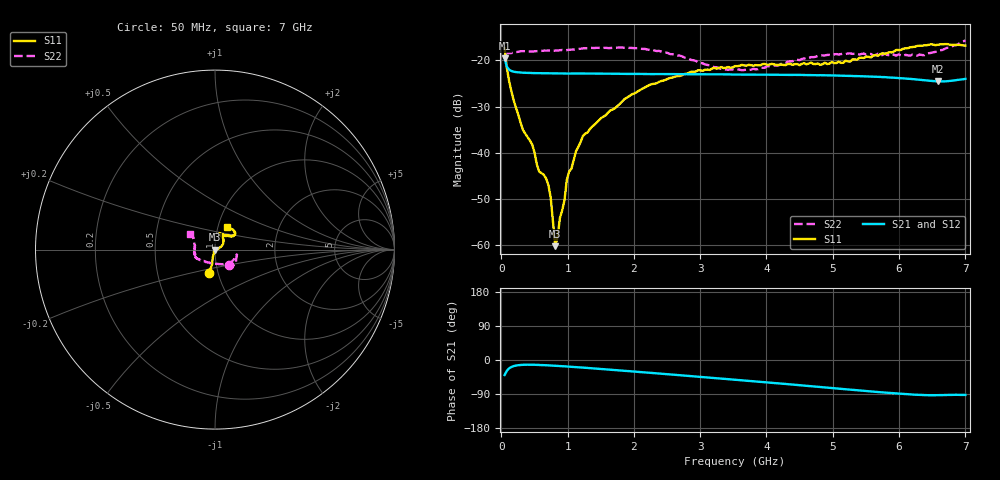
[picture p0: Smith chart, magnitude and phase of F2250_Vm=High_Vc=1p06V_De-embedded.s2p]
! Integrated Device Technology
! Corporate Headquarters
! 6024 Silver Creek Valley Road
! San Jose, CA 95138  USA
! Phone:  1-408-284-8200
! Toll Free:  1-800-223-1366
! Webpage:  http://www.idt.com/
! Timing and RF Division
! 515 Groton Road, Suite 102
! Westford, MA 01886-6024
! Device:  F2250
! Description: Voltage Variable RF Attenuator
! Frequency:  50.0 -  6000.00 MHz
! Package:  3x3 mm Thin QFN Plastic Package: 16 pin
! Ports:  2 RF, 3 DC
!  Pin  1  = GND
!  Pin  2  = NC
!  Pin  3  = RF1  = Port 1
!  Pin  4  = NC
!  Pin  5  = GND
!  Pin  6  = GND
!  Pin  7  = GND
!  Pin  8  = GND
!  Pin  9  = NC
!  Pin 10  = RF2  = Port 2
!  Pin 11  = NC
!  Pin 12  = GND
!  Pin 13  = GND
!  Pin 14  = VCNTRL
!  Pin 15  = VDD
!  Pin 16  = VMODE
! Vcntrl:  1.060 Volts
! Vmode:  +3.300 Volts
! Vdd:  +3.30  Volts
! Current:  1.329 mA
! Data:  The device was measured on a the F2250 evaluation board which has
!  individual transmission lines to the RF pins.  Data was collected
!  using a calibrated network analyzer.  The evaluation board was
!  de-embedded using a TRL calibration technique.
!  The reference plane is the edge of the package pin.
! Misc:  SN 10
!  Action Tracker AT0258
! Date Measured:  2014-11-26
! Date:  2015-10-15  MJV
! Note:
!  Integrated Device Technology supplies this data as a sample of measured
!  data at the package pin for this product.  Your particular data for this
!  product may vary.
!  Data was taken at 25 degrees C.
!  Integrated Device Technology reserves the right to change this data at anytime.
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# GHz S dB R 50
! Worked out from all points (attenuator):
!   201 points, 50 MHz to 7 GHz, reference 50 ohm
!   highest |S21| = -19.60 dB at 50 MHz (marker M1); lowest = -24.6 dB at 6.583 GHz (marker M2)
!   lowest |S11| = -60.2 dB at 814.5 MHz (marker M3), VSWR 1.00, Z = 50 - j0.0982 ohm
!   |S11| at or under -10 dB: start of sweep to end of sweep
!   |S22| runs from -22.2 to -15.7 dB; largest |S21 - S12| = 0.00029
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0.05  -17.37 -104.3  -19.60 -39.6  -19.60 -39.6  -18.87 -48.0
0.1195  -24.60 -103.5  -22.03 -21.8  -22.03 -21.8  -18.44 -18.2
0.29325  -33.58 -105.8  -22.64 -13.1  -22.63 -13.1  -18.03 -13.5
0.467  -38.21 -116.0  -22.75 -12.5  -22.74 -12.5  -18.09 -14.2
0.57125  -44.04 -115.3  -22.77 -13.0  -22.78 -13.1  -18.01 -16.4
0.71025  -46.92 -104.7  -22.80 -14.2  -22.79 -14.2  -17.89 -19.2
0.745  -49.63 -99.7  -22.81 -14.5  -22.80 -14.5  -17.87 -19.8
0.8145  -60.15 -88.2  -22.81 -15.2  -22.81 -15.2  -17.91 -21.5
0.84925  -58.21 -63.9  -22.83 -15.6  -22.83 -15.6  -17.87 -22.5
0.884  -54.07 -27.5  -22.83 -16.0  -22.83 -16.0  -17.82 -23.5
0.9535  -50.19 -37.4  -22.83 -16.7  -22.83 -16.7  -17.85 -24.6
0.98825  -45.83 -23.7  -22.84 -17.1  -22.85 -17.1  -17.79 -25.1
1.12725  -39.62 2.4  -22.84 -18.7  -22.83 -18.7  -17.57 -27.4
1.2315  -36.34 8.4  -22.83 -20.1  -22.84 -20.1  -17.41 -29.5
1.857  -28.38 26.6  -22.93 -28.5  -22.91 -28.5  -17.26 -37.3
2.37825  -24.67 38.1  -22.96 -35.7  -22.96 -35.7  -17.95 -44.1
2.969  -22.15 54.0  -23.01 -44.0  -22.99 -44.1  -20.40 -59.2
3.525  -21.24 67.7  -23.07 -52.1  -23.05 -52.1  -22.05 -93.9
4.7065  -20.79 70.0  -23.19 -69.7  -23.21 -69.6  -19.32 -150.6
5.85325  -18.23 38.5  -23.71 -86.9  -23.70 -87.1  -18.89 -173.0
6.583  -16.64 43.4  -24.55 -92.8  -24.54 -92.9  -17.99 158.0
7  -16.81 61.9  -24.00 -92.3  -23.98 -92.5  -15.70 147.7
